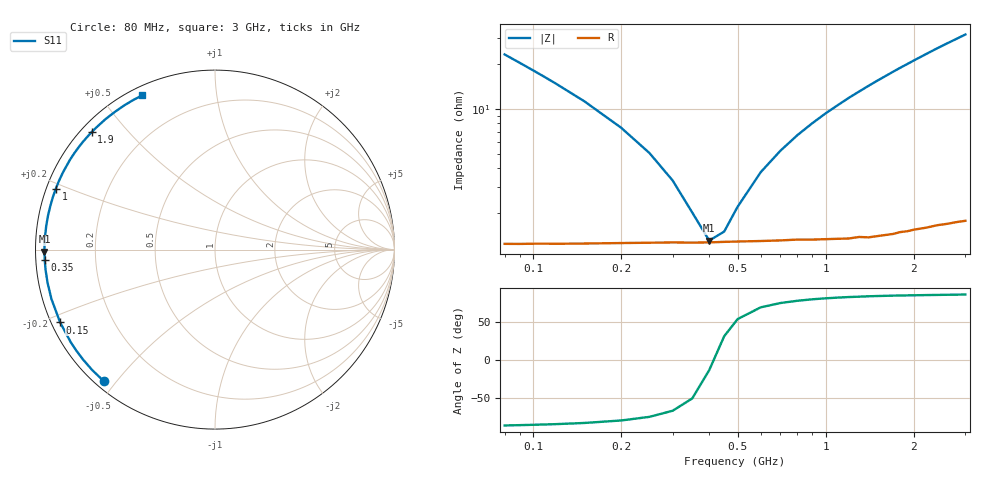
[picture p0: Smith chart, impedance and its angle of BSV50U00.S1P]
! SIEMENS Small Signal Semiconductors
! BB640
! Si Tuning Diode in SOD323
! VR = 0.5 V
! S-Parameters:  July  1993
# GHz  S  MA  R  50
!  f  S11
! GHz  MAG  ANG
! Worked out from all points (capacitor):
!   33 points, 80 MHz to 3 GHz, reference 50 ohm
!   read as one part to ground: C = 82.6 pF near 80 MHz
!   lowest |Z| = 1.31 ohm at 400 MHz (marker M1)
!   series resonance near 414 MHz, so ESL is about 1.8 nH
!   S11 on the Smith chart (normalised r, x): 80 MHz: 0.02, -0.46; 150 MHz: 0.02, -0.22; 350 MHz: 0.03, -0.03; 1 GHz: 0.03, +0.19; 1.9 GHz: 0.03, +0.40; 3 GHz: 0.04, +0.63
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0.08  0.9599 -130.2
0.09  0.9583 -135.6
0.1  0.9569 -140.1
0.11  0.9559 -143.9
0.12  0.9552 -147.2
0.15  0.9535 -154.8
0.2  0.9519 -163.2
0.25  0.9511 -168.8
0.3  0.9506 -173.0
0.35  0.9506 -176.4
0.4  0.9504 -179.3
0.45  0.95 178.2
0.5  0.9498 175.9
0.6  0.9496 171.9
0.7  0.9494 168.4
0.9  0.9495 162.0
1  0.9496 159.0
1.2  0.9501 153.4
1.4  0.9504 148.2
1.6  0.9499 143.3
1.7  0.9498 140.9
1.9  0.9492 136.4
2  0.9488 134.2
2.2  0.9489 130.0
2.4  0.9487 126.0
2.6  0.9493 122.3
2.8  0.9497 118.8
3  0.9505 115.4
